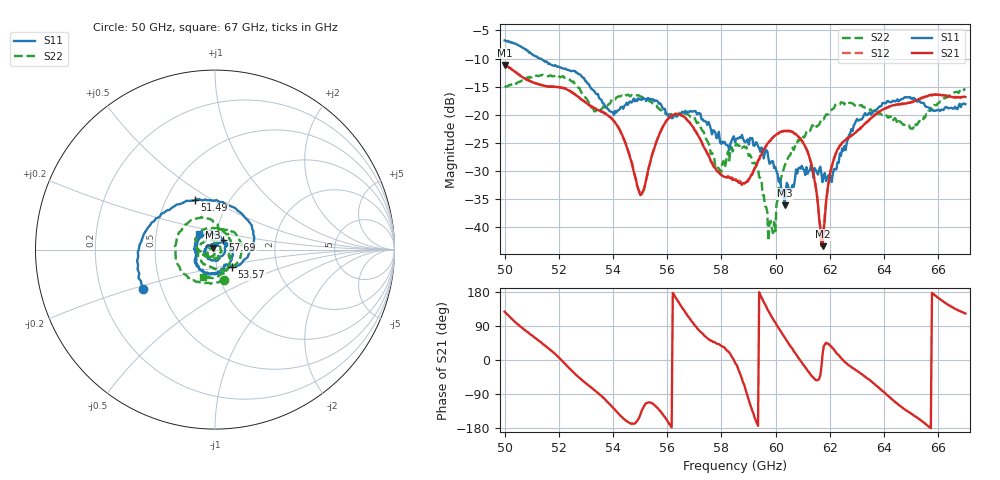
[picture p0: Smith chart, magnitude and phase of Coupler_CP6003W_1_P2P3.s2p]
!Agilent Technologies,E8361A,US42410132,A.06.03.05
!Agilent E8361A: A.06.03.05
!Date: Friday, July 11, 2008 16:29:33
!Correction: S11(Full 2 Port(1,2)) S21(Full 2 Port(1,2)) S12(Full 2 Port(1,2)) S22(Full 2 Port(1,2))
!S2P File: Measurements: S11, S21, S12, S22:
# Hz S  MA  R 50
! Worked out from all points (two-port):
!   401 points, 50 GHz to 67 GHz, reference 50 ohm
!   highest |S21| = -11.17 dB at 50 GHz (marker M1); lowest = -43.4 dB at 61.73 GHz (marker M2)
!   |S21| within 3 dB of the highest: start of sweep to 51 GHz
!   lowest |S11| = -36.2 dB at 60.33 GHz (marker M3), VSWR 1.03, Z = 48.8 + j0.983 ohm
!   |S11| at or under -10 dB: 51.28 GHz to end of sweep
!   |S22| runs from -42.5 to -12.9 dB; largest |S21 - S12| = 0.0052
!   S11 on the Smith chart (normalised r, x): 50 GHz: 0.39, -0.22; 51.49 GHz: 0.70, +0.42; 53.57 GHz: 1.19, -0.23; 57.69 GHz: 1.09, +0.12; 67 GHz: 0.82, +0.14
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5e10  0.458 -151.4  0.2765 127.4  0.2801 127.6  0.1796 -72.9
5.14875e10  0.2961 112.1  0.1798 38.3  0.1808 38.4  0.2226 -169.6
5.28475e10  0.2187 10.1  0.1364 -52.5  0.1359 -52.6  0.1557 94.0
5.357e10  0.1357 -45.0  0.1058 -94.5  0.1073 -94.9  0.1123 74.1
5.425e10  0.1122 -64.6  0.07306 -145.1  0.0732 -145.2  0.1452 35.2
5.5015e10  0.136 -106.7  0.01916 -142.5  0.01943 -143.4  0.1442 -30.0
5.5695e10  0.1251 -152.3  0.06528 -131.3  0.06614 -130.1  0.114 -82.2
5.65875e10  0.1056 169.2  0.09667 134.0  0.09661 134.2  0.098 -140.6
5.76925e10  0.07253 50.8  0.03513 47.3  0.03605 48.7  0.04382 73.1
5.7905e10  0.07028 17.3  0.03092 41.8  0.03071 41.4  0.03308 29.6
5.85e10  0.05695 -88.3  0.02648 -7.5  0.0259 -5.0  0.05071 -96.0
5.9265e10  0.0567 177.2  0.03475 -159.1  0.03548 -158.6  0.03657 -177.7
5.98175e10  0.0372 140.8  0.05883 118.9  0.05947 119.2  0.01129 -170.7
6.03275e10  0.01552 139.6  0.07204 59.7  0.07226 60.4  0.03481 -107.7
6.13475e10  0.03369 96.9  0.03344 -43.9  0.03374 -43.3  0.08033 -162.4
6.173e10  0.02503 57.8  0.006725 14.4  0.006993 12.4  0.09195 -176.8
6.1985e10  0.02934 61.9  0.02733 39.5  0.02732 40.8  0.1053 169.3
6.22825e10  0.03759 74.9  0.04893 15.0  0.04849 16.3  0.1244 149.3
6.29625e10  0.08754 20.8  0.06949 -27.3  0.07015 -27.7  0.1221 95.6
6.4195e10  0.1294 -64.4  0.1183 -97.8  0.1183 -97.5  0.09663 18.5
6.50025e10  0.1386 -119.0  0.1292 -141.8  0.1288 -141.5  0.07525 -13.2
6.7e10  0.1239 137.1  0.1436 122.9  0.1436 122.8  0.1696 -113.9
